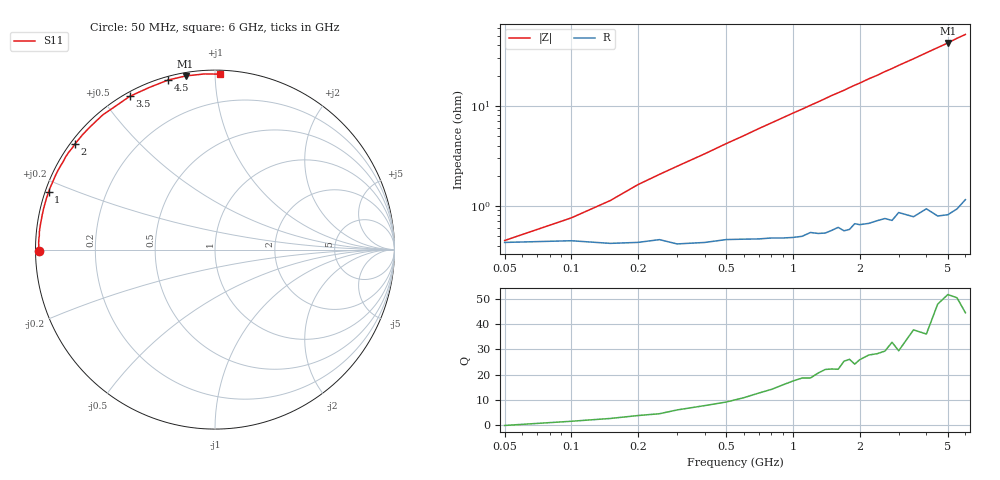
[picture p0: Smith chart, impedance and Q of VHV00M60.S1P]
! Infineon Technologies  Discrete & RF Semiconductors
! BB 814
! Si Tuning Diode in SOT23
! VR =
! S-Parameters:  July  1999
# GHz  S  MA  R  50
!  f  S11
! GHz  MAG  ANG
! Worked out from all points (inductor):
!   34 points, 50 MHz to 6 GHz, reference 50 ohm
!   read as one part to ground: L = 1.28 nH near 200 MHz
!   highest Q = 50.6 at 5 GHz (marker M1), where L = 1.34 nH
!   S11 on the Smith chart (normalised r, x): 50 MHz: 0.01, -0.00; 1 GHz: 0.01, +0.17; 2 GHz: 0.01, +0.34; 3.5 GHz: 0.02, +0.59; 4.5 GHz: 0.02, +0.76; 6 GHz: 0.02, +1.03
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0.05  0.9829 -179.7
0.1  0.9823 178.6
0.15  0.9833 177.6
0.2  0.9829 176.4
0.3  0.9835 174.4
0.4  0.983 172.5
0.6  0.9818 168.6
0.8  0.9814 164.7
1  0.9814 160.9
1.1  0.981 159.1
1.3  0.98 155.4
1.5  0.9788 151.6
1.6  0.9776 149.9
1.7  0.9794 148.2
1.8  0.9789 146.3
1.9  0.9762 144.5
2  0.977 142.9
2.2  0.9768 139.3
2.4  0.9758 136.2
2.6  0.9753 132.7
2.8  0.9769 129.7
3  0.9731 126.4
3.5  0.9772 119.1
4  0.9747 112.0
4.5  0.9802 105.5
5  0.9812 99.6
5.5  0.9805 93.4
6  0.9779 88.4
